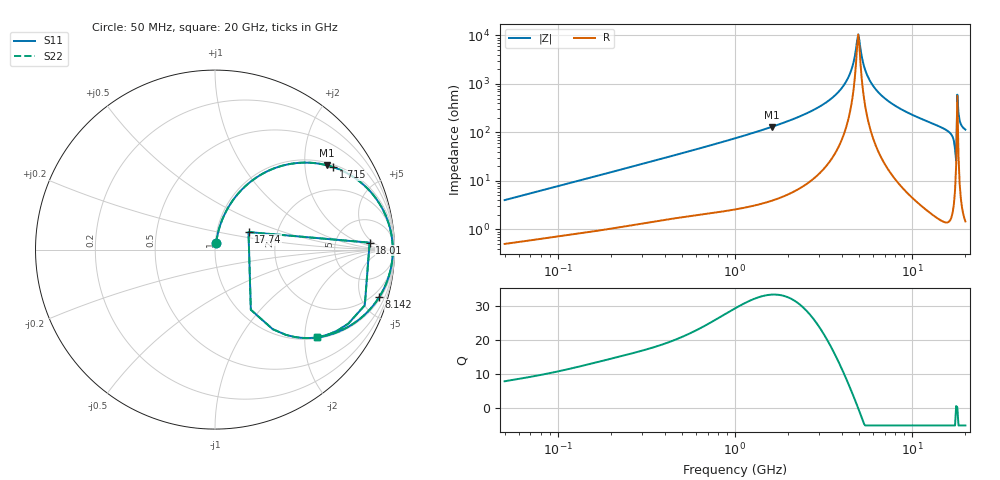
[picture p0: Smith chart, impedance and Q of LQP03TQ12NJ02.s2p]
!Murata Part Number: LQP03TQ12NJ02
!These Parameters are Measured in Series Mode Connection
!  o--[Z]--o
!Port1  Port2
!  o-------o
!Freq. Start=50[MHz] Stop=20[GHz], 401[Steps]
# Hz S RI R 50
!Freq.(Hz) S11(Real) S11(Imag) S21(Real) S21(Imag) S12(Real) S12(Imag) S22(Real) S22(Imag)
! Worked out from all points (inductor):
!   401 points, 50 MHz to 20 GHz, reference 50 ohm
!   read as one part in series: L = 12.5 nH near 51.52 MHz
!   highest Q = 33.3 at 1.615 GHz (marker M1), where L = 12.8 nH
!   self-resonance near 4.893 GHz
!   S11 on the Smith chart (normalised r, x): 50 MHz: 1.01, +0.08; 1.715 GHz: 1.08, +2.81; 8.142 GHz: 1.20, -6.87; 17.74 GHz: 1.42, +0.29; 18.01 GHz: 12, +4; 20 GHz: 1.03, -2.29
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5e7  0.00655 0.0394  0.9935 -0.0394  0.9935 -0.0394  0.00655 0.0394
1.364002e8  0.0188 0.1015  0.9812 -0.1015  0.9812 -0.1015  0.0188 0.1015
3.721004e8  0.083 0.2501  0.917 -0.2501  0.917 -0.2501  0.083 0.2501
1e9  0.3674 0.4653  0.6326 -0.4653  0.6326 -0.4653  0.3674 0.4653
1.614971e9  0.6255 0.4692  0.3745 -0.4692  0.3745 -0.4692  0.6255 0.4692
1.714689e9  0.6588 0.4594  0.3412 -0.4594  0.3412 -0.4594  0.6588 0.4594
2.728004e9  0.8786 0.3084  0.1214 -0.3084  0.1214 -0.3084  0.8786 0.3084
4.087748e9  0.9782 0.1063  0.0218 -0.1063  0.0218 -0.1063  0.9782 0.1063
4.539627e9  0.9878 0.0494  0.0122 -0.0494  0.0122 -0.0494  0.9878 0.0494
4.966507e9  0.9905 -1.46e-05  0.00946 1.46e-05  0.00946 1.46e-05  0.9905 -1.46e-05
5.433528e9  0.9883 -0.0495  0.0117 0.0495  0.0117 0.0495  0.9883 -0.0495
5.769027e9  0.9841 -0.0824  0.0159 0.0824  0.0159 0.0824  0.9841 -0.0824
7.442007e9  0.9406 -0.2186  0.0594 0.2186  0.0594 0.2186  0.9406 -0.2186
8.141811e9  0.9154 -0.264  0.0846 0.264  0.0846 0.264  0.9154 -0.264
1.621653e10  0.5045 -0.4928  0.4955 0.4928  0.4955 0.4928  0.5045 -0.4928
1.696185e10  0.3953 -0.4751  0.6047 0.4751  0.6047 0.4751  0.3953 -0.4751
1.721783e10  0.3215 -0.4433  0.6785 0.4433  0.6785 0.4433  0.3215 -0.4433
1.774144e10  0.1867 0.0977  0.8133 -0.0977  0.8133 -0.0977  0.1867 0.0977
1.800918e10  0.8616 0.0386  0.1384 -0.0386  0.1384 -0.0386  0.8616 0.0386
1.855685e10  0.743 -0.4122  0.257 0.4122  0.257 0.4122  0.743 -0.4122
1.912117e10  0.6416 -0.4689  0.3584 0.4689  0.3584 0.4689  0.6416 -0.4689
2e10  0.5656 -0.4893  0.4344 0.4893  0.4344 0.4893  0.5656 -0.4893
